INTERFACE ITF_Axis



METHOD M_MoveVel : BOOL
VAR_INPUT
	Execute:BOOL;
END_VAR
END_METHOD

METHOD M_PowerOff : BOOL
VAR_INPUT

END_VAR
END_METHOD

METHOD M_PowerOn : BOOL
VAR_INPUT

END_VAR
END_METHOD

METHOD M_Stop : BOOL
VAR_INPUT
	Execute:BOOL;
END_VAR
END_METHOD

PROPERTY P_Status : ST_AxisStatus
GET
END_GET
END_PROPERTY

END_INTERFACE
